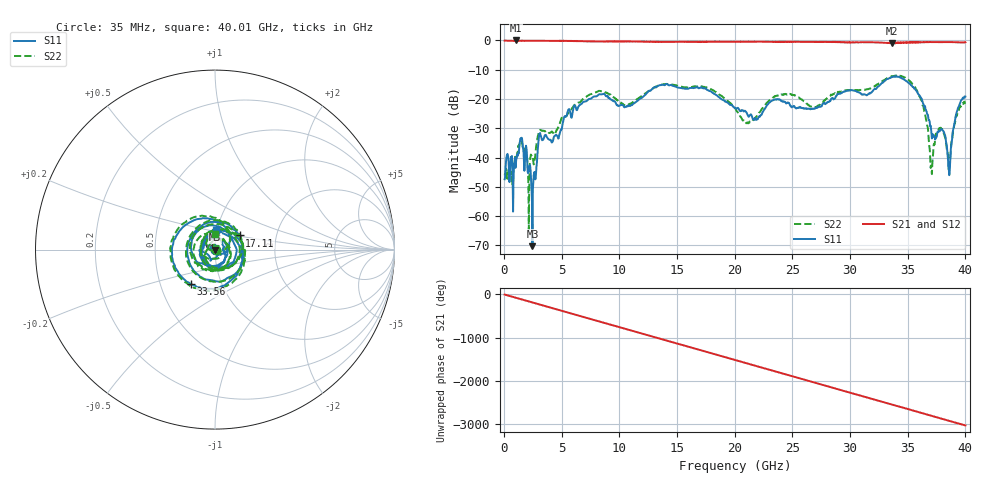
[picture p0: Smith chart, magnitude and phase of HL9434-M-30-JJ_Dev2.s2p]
! 5/27/2020 7:41:22 AM
! H:\PRODUCTION_DATA\TEMP_S2P.S2P
! CHANNEL.1
! TR.MEASUREMENT
! CORRECTED.DATA
# GHZ S RI R 50.0
! FREQ.GHZ  S11RE  S11IM  S21RE  S21IM  S12RE  S12IM  S22RE  S22IM
!; PortSelection: Port_12
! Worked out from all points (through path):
!   1143 points, 35 MHz to 40.01 GHz, reference 50 ohm
!   highest |S21| = 0.01 dB at 1.05 GHz (marker M1); lowest = -1.0 dB at 33.67 GHz (marker M2)
!   group delay of S21, straight-line fit = 210 ps
!   lowest |S11| = -70.2 dB at 2.45 GHz (marker M3), VSWR 1.00, Z = 50 - j0.0126 ohm
!   |S11| at or under -10 dB: start of sweep to end of sweep
!   |S22| runs from -64.6 to -12.0 dB; largest |S21 - S12| = 0.037
!   S11 on the Smith chart (normalised r, x): 35 MHz: 1.01, -0.00; 17.11 GHz: 1.30, +0.21; 33.56 GHz: 0.71, -0.29; 40.01 GHz: 0.98, +0.22
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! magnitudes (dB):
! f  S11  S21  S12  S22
! 35 MHz  -47.4  0.0  0.0  -46.1
! 1.05 GHz  -40.4  0.0  -0.1  -39.0
! 1.505 GHz  -33.2  -0.1  -0.1  -34.4
! 2.03 GHz  -44.6  -0.1  -0.1  -42.7
! 2.45 GHz  -70.2  -0.1  -0.1  -39.5
! 3.115 GHz  -31.6  -0.1  -0.1  -30.5
! 6.72 GHz  -21.6  -0.3  -0.2  -20.5
! 13.37 GHz  -15.4  -0.5  -0.4  -15.3
! 17.11 GHz  -16.0  -0.4  -0.5  -15.8
! 20.02 GHz  -23.0  -0.4  -0.4  -23.1
! 21.18 GHz  -25.9  -0.4  -0.4  -28.3
! 23.7 GHz  -20.0  -0.4  -0.5  -18.8
! 26.7 GHz  -23.3  -0.5  -0.5  -22.7
! 33.35 GHz  -13.0  -0.9  -0.8  -12.6
! 33.56 GHz  -12.6  -0.9  -0.8  -12.3
! 33.67 GHz  -12.5  -1.0  -0.7  -12.2
! 35.95 GHz  -18.4  -0.7  -0.5  -18.0
! 37.06 GHz  -32.1  -0.5  -0.5  -44.1
! 37.84 GHz  -30.6  -0.6  -0.6  -29.8
! 38.6 GHz  -46.0  -0.5  -0.5  -43.4
! 39.23 GHz  -24.6  -0.6  -0.6  -25.6
! 40.01 GHz  -19.2  -0.6  -0.7  -21.3
